|   IBIS model for TI xxx DSP
[IBIS Ver]   5.1
[Disclaimer]   Please be aware that in the absence of a written agreement
|   Texas Instruments(TI) assumes no liability for:
|   (1) The accuracy of the IBIS models provided to your company,
|   however, the IBIS model is compliant to industry standard
|   IQ Level 2a.  Refer to IBIS Quality Section below for
|   for full details.
|   (2) The proper functioning of these Models in your design
|   or for any resulting applications
|   (3) Infringement of patents, copyrights or intellectual
|   property rights resulting from your use of these
|   models.
|   TI provides IBIS Models as a service to our customers and
|   therefore reserves the right to limit distribution of the
|   Models.  The information is subject to change without notice.
[File Name]  j742s2.ibs
[File Rev]   0.1
|   -Initial version
[Date]   28 March 2024
[Source]   Texas Instruments Incorporated
[Copyright]   Property of Texas Instruments Incorporated.
|   Unauthorized reproduction and/or distribution is strictly.
|   prohibited.
|   This product is protected under copyright law and trade
|   secret law as an unpublished work.
|   Created 2012,(C) Copyright 1999-2012,
|   Texas Instruments Incorporated., All Rights Reserved.
|   These commodities are under the U.S. Government
|   distribution license control. As such,they are not to be
|   re-exported without the prior approval of the U.S.
|   Department of Commerce.
[Notes]
|   This file does not include AMI models for the following:
|   1. PCIe
|   2. CSI
|   3. Display Port
|   4. USB2
|   5. USB3
|   6. MPHY
|   For SerDes simulations use Texas Instruments IBIS AMI models
|   Some IV curves contain Non monotonic data points.
|   Revision History
|   GERNERAL COMMENT: All IBIS Quality Notes below reflect latest release
|   and version of IBIS File
|   File passes ibischk6 and ibischk7 with 0 errors and 91 warnings
|   v0.1: Initial version
|   Component j742s2
[Component] j742s2
[Manufacturer] Texas Instruments
[Package]
|   typ   min   max
R_pkg   0.61008   0.049437   1.2542
L_pkg   3.63e-9   6.144e-10   6.964e-9
C_pkg   1.799e-12   7.984e-13   3.865e-12
[Pin]	Signal_name	model_name
M30	ATEST0	NC
J29	ATEST1	NC
T27	CAP_VDDS0	POWER
J25	CAP_VDDS0_MCU	POWER
J23	CAP_VDDS1_MCU	POWER
P27	CAP_VDDS2	POWER
J24	CAP_VDDS2_MCU	POWER
M27	CAP_VDDS5	POWER
AH33	CSI0_RXCLKN	NC
AH32	CSI0_RXCLKP	NC
AL32	CSI0_RXN0	NC
AM31	CSI0_RXN1	NC
AN30	CSI0_RXN2	NC
AK33	CSI0_RXN3	NC
AL31	CSI0_RXP0	NC
AM30	CSI0_RXP1	NC
AN29	CSI0_RXP2	NC
AK32	CSI0_RXP3	NC
AH31	CSI0_RXRCALIB	NC
AE29	CSI1_RXCLKN	NC
AF29	CSI1_RXCLKP	NC
AF30	CSI1_RXN0	NC
AE33	CSI1_RXN1	NC
AE31	CSI1_RXN2	NC
AF32	CSI1_RXN3	NC
AG30	CSI1_RXP0	NC
AF33	CSI1_RXP1	NC
AF31	CSI1_RXP2	NC
AG32	CSI1_RXP3	NC
AJ33	CSI1_RXRCALIB	NC
AC29	CSI2_RXCLKN	NC
AB29	CSI2_RXCLKP	NC
AC30	CSI2_RXN0	NC
AB31	CSI2_RXN1	NC
AC32	CSI2_RXN2	NC
AB33	CSI2_RXN3	NC
AD30	CSI2_RXP0	NC
AC31	CSI2_RXP1	NC
AD32	CSI2_RXP2	NC
AC33	CSI2_RXP3	NC
AH29	CSI2_RXRCALIB	NC
AA3	DDR0_CA0	DDR_SE
Y4	DDR0_CA1	DDR_SE
AA4	DDR0_CA2	DDR_SE
AB3	DDR0_CA3	DDR_SE
Y3	DDR0_CA4	DDR_SE
AB5	DDR0_CA5	DDR_SE
R7	DDR0_CAL0	DDR_SE
AB6	DDR0_CKE0	DDR_SE
AB7	DDR0_CKE1	DDR_SE
Y2	DDR0_CKN	DDR_DIFF
AA1	DDR0_CKP	DDR_DIFF
AA6	DDR0_CSN0_0	DDR_SE
Y5	DDR0_CSN0_1	DDR_SE
Y7	DDR0_CSN1_0	DDR_SE
AA7	DDR0_CSN1_1	DDR_SE
U6	DDR0_DM0	DDR_SE
V2	DDR0_DM1	DDR_SE
AE2	DDR0_DM2	DDR_SE
AF6	DDR0_DM3	DDR_SE
R5	DDR0_DQ0	DDR_SE
R4	DDR0_DQ1	DDR_SE
W3	DDR0_DQ10	DDR_SE
V5	DDR0_DQ11	DDR_SE
W6	DDR0_DQ12	DDR_SE
U2	DDR0_DQ13	DDR_SE
W4	DDR0_DQ14	DDR_SE
U3	DDR0_DQ15	DDR_SE
AD5	DDR0_DQ16	DDR_SE
AC3	DDR0_DQ17	DDR_SE
AE3	DDR0_DQ18	DDR_SE
AB2	DDR0_DQ19	DDR_SE
R2	DDR0_DQ2	DDR_SE
AC4	DDR0_DQ20	DDR_SE
AD2	DDR0_DQ21	DDR_SE
AC6	DDR0_DQ22	DDR_SE
AD4	DDR0_DQ23	DDR_SE
AG4	DDR0_DQ24	DDR_SE
AG2	DDR0_DQ25	DDR_SE
AF3	DDR0_DQ26	DDR_SE
AE5	DDR0_DQ27	DDR_SE
AE6	DDR0_DQ28	DDR_SE
AG5	DDR0_DQ29	DDR_SE
T4	DDR0_DQ3	DDR_SE
AF4	DDR0_DQ30	DDR_SE
AH6	DDR0_DQ31	DDR_SE
U5	DDR0_DQ4	DDR_SE
T3	DDR0_DQ5	DDR_SE
T6	DDR0_DQ6	DDR_SE
T7	DDR0_DQ7	DDR_SE
V4	DDR0_DQ8	DDR_SE
V7	DDR0_DQ9	DDR_SE
T1	DDR0_DQS0N	DDR_DIFF
R1	DDR0_DQS0P	DDR_DIFF
W1	DDR0_DQS1N	DDR_DIFF
V1	DDR0_DQS1P	DDR_DIFF
AC1	DDR0_DQS2N	DDR_DIFF
AD1	DDR0_DQS2P	DDR_DIFF
AF1	DDR0_DQS3N	DDR_DIFF
AG1	DDR0_DQS3P	DDR_DIFF
W7	DDR0_RESETN	DDR_SE
AC7	DDR0_RET	DDR_SE
J4	DDR1_CA0	DDR_SE
H3	DDR1_CA1	DDR_SE
G2	DDR1_CA2	DDR_SE
J3	DDR1_CA3	DDR_SE
G3	DDR1_CA4	DDR_SE
H4	DDR1_CA5	DDR_SE
F8	DDR1_CAL0	DDR_SE
E7	DDR1_CKE0	DDR_SE
H6	DDR1_CKE1	DDR_SE
H1	DDR1_CKN	DDR_DIFF
J2	DDR1_CKP	DDR_DIFF
G6	DDR1_CSN0_0	DDR_SE
G7	DDR1_CSN0_1	DDR_SE
H7	DDR1_CSN1_0	DDR_SE
F6	DDR1_CSN1_1	DDR_SE
A3	DDR1_DM0	DDR_SE
F3	DDR1_DM1	DDR_SE
L2	DDR1_DM2	DDR_SE
P2	DDR1_DM3	DDR_SE
A6	DDR1_DQ0	DDR_SE
C6	DDR1_DQ1	DDR_SE
E2	DDR1_DQ10	DDR_SE
F4	DDR1_DQ11	DDR_SE
D6	DDR1_DQ12	DDR_SE
E4	DDR1_DQ13	DDR_SE
D3	DDR1_DQ14	DDR_SE
D5	DDR1_DQ15	DDR_SE
M3	DDR1_DQ16	DDR_SE
K4	DDR1_DQ17	DDR_SE
M2	DDR1_DQ18	DDR_SE
L5	DDR1_DQ19	DDR_SE
A5	DDR1_DQ2	DDR_SE
J5	DDR1_DQ20	DDR_SE
K3	DDR1_DQ21	DDR_SE
L4	DDR1_DQ22	DDR_SE
K6	DDR1_DQ23	DDR_SE
N6	DDR1_DQ24	DDR_SE
P4	DDR1_DQ25	DDR_SE
N3	DDR1_DQ26	DDR_SE
M5	DDR1_DQ27	DDR_SE
M6	DDR1_DQ28	DDR_SE
P5	DDR1_DQ29	DDR_SE
C4	DDR1_DQ3	DDR_SE
N4	DDR1_DQ30	DDR_SE
P6	DDR1_DQ31	DDR_SE
B4	DDR1_DQ4	DDR_SE
B2	DDR1_DQ5	DDR_SE
C3	DDR1_DQ6	DDR_SE
B5	DDR1_DQ7	DDR_SE
E5	DDR1_DQ8	DDR_SE
D2	DDR1_DQ9	DDR_SE
C1	DDR1_DQS0N	DDR_DIFF
B1	DDR1_DQS0P	DDR_DIFF
F1	DDR1_DQS1N	DDR_DIFF
E1	DDR1_DQS1P	DDR_DIFF
K1	DDR1_DQS2N	DDR_DIFF
L1	DDR1_DQS2P	DDR_DIFF
N1	DDR1_DQS3N	DDR_DIFF
P1	DDR1_DQS3P	DDR_DIFF
G5	DDR1_RESETN	DDR_SE
G8	DDR1_RET	DDR_SE
AJ25	DP0_AUXN	NC
AJ24	DP0_AUXP	NC
AJ28	DSI0_TXCLKN	NC
AJ27	DSI0_TXCLKP	NC
AL26	DSI0_TXN0	NC
AK27	DSI0_TXN1	NC
AM25	DSI0_TXN2	NC
AN24	DSI0_TXN3	NC
AL25	DSI0_TXP0	NC
AK26	DSI0_TXP1	NC
AM24	DSI0_TXP2	NC
AN23	DSI0_TXP3	NC
AH25	DSI0_TXRCALIB	NC
AJ31	DSI1_TXCLKN	NC
AJ30	DSI1_TXCLKP	NC
AK30	DSI1_TXN0	NC
AL29	DSI1_TXN1	NC
AM28	DSI1_TXN2	NC
AN27	DSI1_TXN3	NC
AK29	DSI1_TXP0	NC
AL28	DSI1_TXP1	NC
AM27	DSI1_TXP2	NC
AN26	DSI1_TXP3	NC
AH27	DSI1_TXRCALIB	NC
L31	ECAP0_IN_APWM_OUT	LVCMOS_H
F19	EMU0	LVCMOS_V
E17	EMU1	LVCMOS_V
J33	EXT_REFCLK1	LVCMOS_H
Y29	EXTINTN	IIC_H
P32	GPIO0_11	LVCMOS_H
E33	GPIO0_12	LVCMOS_H
AA30	I2C0_SCL	IIC_H
Y30	I2C0_SDA	IIC_H
L30	IFORCE	NC
AH7	LJCB_DUAL_ATEST0	NC
AH8	LJCB_DUAL_ATEST1	NC
L28	MAIN_ATEST	NC
G29	MCAN0_RX	LVCMOS_H
N33	MCAN0_TX	LVCMOS_H
H31	MCAN1_RX	LVCMOS_H
G33	MCAN1_TX	LVCMOS_H
T29	MCAN12_RX	LVCMOS_H
P29	MCAN12_TX	LVCMOS_H
T32	MCAN13_RX	LVCMOS_H
T31	MCAN13_TX	LVCMOS_H
R30	MCAN14_RX	LVCMOS_H
R33	MCAN14_TX	LVCMOS_H
R31	MCAN15_RX	LVCMOS_H
R29	MCAN15_TX	LVCMOS_H
U30	MCAN16_RX	LVCMOS_H
G30	MCAN16_TX	LVCMOS_H
F33	MCAN2_RX	LVCMOS_H
G28	MCAN2_TX	LVCMOS_H
J30	MCASP0_ACLKX	LVCMOS_H
K31	MCASP0_AFSX	LVCMOS_H
F32	MCASP0_AXR0	LVCMOS_H
H32	MCASP0_AXR1	LVCMOS_H
L32	MCASP0_AXR10	LVCMOS_H
P30	MCASP0_AXR11	LVCMOS_H
M32	MCASP0_AXR12	LVCMOS_H
L33	MCASP0_AXR13	LVCMOS_H
U31	MCASP0_AXR14	LVCMOS_H
M33	MCASP0_AXR15	LVCMOS_H
H33	MCASP0_AXR2	LVCMOS_H
F31	MCASP0_AXR3	LVCMOS_H
J32	MCASP0_AXR4	LVCMOS_H
H30	MCASP0_AXR5	LVCMOS_H
K33	MCASP0_AXR6	LVCMOS_H
M31	MCASP0_AXR7	LVCMOS_H
N30	MCASP0_AXR8	LVCMOS_H
T33	MCASP0_AXR9	LVCMOS_H
U32	MCASP1_ACLKX	LVCMOS_H
N32	MCASP1_AFSX	LVCMOS_H
H29	MCASP1_AXR0	LVCMOS_H
G31	MCASP1_AXR1	LVCMOS_H
J31	MCASP1_AXR2	LVCMOS_H
P31	MCASP1_AXR3	LVCMOS_H
N31	MCASP1_AXR4	LVCMOS_H
P33	MCASP2_ACLKX	LVCMOS_H
G32	MCASP2_AFSX	LVCMOS_H
K32	MCASP2_AXR0	LVCMOS_H
R32	MCASP2_AXR1	LVCMOS_H
E26	MCU_ADC0_AIN0	NC
F25	MCU_ADC0_AIN1	NC
F23	MCU_ADC0_AIN2	NC
A28	MCU_ADC0_AIN3	NC
E24	MCU_ADC0_AIN4	NC
D27	MCU_ADC0_AIN5	NC
A26	MCU_ADC0_AIN6	NC
B27	MCU_ADC0_AIN7	NC
C26	MCU_ADC0_REFN	NC
D25	MCU_ADC0_REFP	NC
C32	MCU_ADC1_AIN0	NC
B33	MCU_ADC1_AIN1	NC
B31	MCU_ADC1_AIN2	NC
B29	MCU_ADC1_AIN3	NC
D31	MCU_ADC1_AIN4	NC
A32	MCU_ADC1_AIN5	NC
A30	MCU_ADC1_AIN6	NC
C28	MCU_ADC1_AIN7	NC
D29	MCU_ADC1_REFN	NC
C30	MCU_ADC1_REFP	NC
D22	MCU_I2C0_SCL	IIC_V
A21	MCU_I2C0_SDA	IIC_V
C18	MCU_MCAN0_RX	LVCMOS_V
E22	MCU_MCAN0_TX	LVCMOS_V
E12	MCU_MDIO0_MDC	LVCMOS_V
F13	MCU_MDIO0_MDIO	LVCMOS_V
D8	MCU_OSPI0_CLK	LVCMOS_V
F12	MCU_OSPI0_CSN0	LVCMOS_V
F11	MCU_OSPI0_CSN1	LVCMOS_V
F10	MCU_OSPI0_CSN2	LVCMOS_V
E11	MCU_OSPI0_CSN3	LVCMOS_V
E10	MCU_OSPI0_D0	LVCMOS_V
F9	MCU_OSPI0_D1	LVCMOS_V
E9	MCU_OSPI0_D2	LVCMOS_V
D11	MCU_OSPI0_D3	LVCMOS_V
D9	MCU_OSPI0_D4	LVCMOS_V
C9	MCU_OSPI0_D5	LVCMOS_V
C7	MCU_OSPI0_D6	LVCMOS_V
C8	MCU_OSPI0_D7	LVCMOS_V
C10	MCU_OSPI0_DQS	LVCMOS_V
D10	MCU_OSPI0_LBCLKO	LVCMOS_V
B7	MCU_OSPI1_CLK	LVCMOS_V
A8	MCU_OSPI1_CSN0	LVCMOS_V
A9	MCU_OSPI1_CSN1	LVCMOS_V
B8	MCU_OSPI1_D0	LVCMOS_V
B11	MCU_OSPI1_D1	LVCMOS_V
A11	MCU_OSPI1_D2	LVCMOS_V
A10	MCU_OSPI1_D3	LVCMOS_V
B9	MCU_OSPI1_DQS	LVCMOS_V
B10	MCU_OSPI1_LBCLKO	LVCMOS_V
C24	MCU_PORZ	RESET_H
E21	MCU_RESETSTATZ	LVCMOS_V
E20	MCU_RESETZ	LVCMOS_V
E13	MCU_RGMII1_RD0	LVCMOS_V
D14	MCU_RGMII1_RD1	LVCMOS_V
D12	MCU_RGMII1_RD2	LVCMOS_V
D13	MCU_RGMII1_RD3	LVCMOS_V
C12	MCU_RGMII1_RX_CTL	LVCMOS_V
C14	MCU_RGMII1_RXC	LVCMOS_V
B13	MCU_RGMII1_TD0	LVCMOS_V
A13	MCU_RGMII1_TD1	LVCMOS_V
B12	MCU_RGMII1_TD2	LVCMOS_V
A12	MCU_RGMII1_TD3	LVCMOS_V
B14	MCU_RGMII1_TX_CTL	LVCMOS_V
A14	MCU_RGMII1_TXC	LVCMOS_V
C22	MCU_SAFETY_ERRORN	LVCMOS_V
F15	MCU_SPI0_CLK	LVCMOS_V
E19	MCU_SPI0_CS0	LVCMOS_V
E18	MCU_SPI0_D0	LVCMOS_V
E14	MCU_SPI0_D1	LVCMOS_V
AH2	MMC0_CALPAD	EMMC
AJ2	MMC0_CLK	EMMC
AL2	MMC0_CMD	EMMC
AM1	MMC0_DAT0	EMMC
AK3	MMC0_DAT1	EMMC
AL1	MMC0_DAT2	EMMC
AK1	MMC0_DAT3	EMMC
AJ3	MMC0_DAT4	EMMC
AH3	MMC0_DAT5	EMMC
AJ4	MMC0_DAT6	EMMC
AK2	MMC0_DAT7	EMMC
AJ1	MMC0_DS	EMMC
AH4	MMC0_VCTRL_TP	EMMC
D33	MMC1_CLK	SDIO_H
E32	MMC1_CMD	SDIO_H
F28	MMC1_DAT0	SDIO_H
F29	MMC1_DAT1	SDIO_H
E30	MMC1_DAT2	SDIO_H
F30	MMC1_DAT3	SDIO_H
B23	OSC1_XI	NC
A22	OSC1_XO	NC
AJ13	PCIE_REFCLK0_N_OUT	NC
AJ12	PCIE_REFCLK0_P_OUT	NC
AH14	PCIE_REFCLK1_N_OUT	NC
AH13	PCIE_REFCLK1_P_OUT	NC
AH11	PCIE_REFCLK2_N_OUT	NC
AH10	PCIE_REFCLK2_P_OUT	NC
AJ16	PCIE_REFCLK3_N_OUT	NC
AJ15	PCIE_REFCLK3_P_OUT	NC
B16	PMIC_POWER_EN1	LVCMOS_V
T30	PMIC_WAKE0	LVCMOS_H
D24	PORZ	RESET_H
G20	RESET_REQZ	LVCMOS_V
W32	RESETSTATZ	LVCMOS_H
AK15	SERDES0_REFCLK_N	NC
AK14	SERDES0_REFCLK_P	NC
AG7	SERDES0_REXT	NC
AM12	SERDES0_RX0_N	NC
AM13	SERDES0_RX0_P	NC
AL13	SERDES0_RX1_N	NC
AL14	SERDES0_RX1_P	NC
AN15	SERDES0_RX2_N	NC
AN14	SERDES0_RX2_P	NC
AL17	SERDES0_RX3_N	NC
AL16	SERDES0_RX3_P	NC
AN11	SERDES0_TX0_N	NC
AN12	SERDES0_TX0_P	NC
AJ19	SERDES0_TX1_N	NC
AJ18	SERDES0_TX1_P	NC
AM16	SERDES0_TX2_N	NC
AM15	SERDES0_TX2_P	NC
AK18	SERDES0_TX3_N	NC
AK17	SERDES0_TX3_P	NC
AN5	SERDES1_REFCLK_N	NC
AN6	SERDES1_REFCLK_P	NC
AH9	SERDES1_REXT	NC
AL10	SERDES1_RX0_N	NC
AL11	SERDES1_RX0_P	NC
AN8	SERDES1_RX1_N	NC
AN9	SERDES1_RX1_P	NC
AM6	SERDES1_RX2_N	NC
AM7	SERDES1_RX2_P	NC
AL7	SERDES1_RX3_N	NC
AL8	SERDES1_RX3_P	NC
AK11	SERDES1_TX0_N	NC
AK12	SERDES1_TX0_P	NC
AM9	SERDES1_TX1_N	NC
AM10	SERDES1_TX1_P	NC
AK8	SERDES1_TX2_N	NC
AK9	SERDES1_TX2_P	NC
AJ9	SERDES1_TX3_N	NC
AJ10	SERDES1_TX3_P	NC
AK21	SERDES4_REFCLK_N	NC
AK20	SERDES4_REFCLK_P	NC
AH23	SERDES4_REXT	NC
AN17	SERDES4_RX0_N	NC
AN18	SERDES4_RX0_P	NC
AL19	SERDES4_RX1_N	NC
AL20	SERDES4_RX1_P	NC
AK23	SERDES4_RX2_N	NC
AK24	SERDES4_RX2_P	NC
AM21	SERDES4_RX3_N	NC
AM22	SERDES4_RX3_P	NC
AJ21	SERDES4_TX0_N	NC
AJ22	SERDES4_TX0_P	NC
AM18	SERDES4_TX1_N	NC
AM19	SERDES4_TX1_P	NC
AN20	SERDES4_TX2_N	NC
AN21	SERDES4_TX2_P	NC
AL22	SERDES4_TX3_N	NC
AL23	SERDES4_TX3_P	NC
Y31	SOC_SAFETY_ERRORN	LVCMOS_H
V31	SPI0_CLK	LVCMOS_H
Y33	SPI0_CS0	LVCMOS_H
Y32	SPI0_CS1	LVCMOS_H
V30	SPI0_D0	LVCMOS_H
W31	SPI0_D1	LVCMOS_H
F21	TCK	LVCMOS_V
V33	TDI	LVCMOS_H
W33	TDO	LVCMOS_H
E28	TEMP_DIODE_P	NC
F27	TEMP_DIODE_P	NC
AA32	TIMER_IO0	LVCMOS_H
W30	TIMER_IO1	LVCMOS_H
V32	TMS	LVCMOS_H
F17	TRSTN	LVCMOS_V
AJ5	UFS0_REF_CLK	NC
AJ7	UFS0_RSTN	NC
AK5	UFS0_RX_DN0	NC
AL4	UFS0_RX_DN1	NC
AK6	UFS0_RX_DP0	NC
AL5	UFS0_RX_DP1	NC
AN2	UFS0_TX_DN0	NC
AM3	UFS0_TX_DN1	NC
AN3	UFS0_TX_DP0	NC
AM4	UFS0_TX_DP1	NC
AH16	USB0_DM	NC
AH17	USB0_DP	NC
AH20	USB0_ID	NC
AH22	USB0_RCALIB	NC
AG19	USB0_VBUS	NC
K9	VDD_CORE	POWER
K11	VDD_CORE	POWER
K15	VDD_CORE	POWER
K17	VDD_CORE	POWER
L10	VDD_CORE	POWER
L12	VDD_CORE	POWER
L14	VDD_CORE	POWER
L16	VDD_CORE	POWER
M9	VDD_CORE	POWER
M11	VDD_CORE	POWER
M13	VDD_CORE	POWER
M15	VDD_CORE	POWER
M17	VDD_CORE	POWER
N10	VDD_CORE	POWER
N12	VDD_CORE	POWER
N14	VDD_CORE	POWER
N16	VDD_CORE	POWER
N22	VDD_CORE	POWER
N24	VDD_CORE	POWER
N26	VDD_CORE	POWER
P9	VDD_CORE	POWER
P11	VDD_CORE	POWER
P25	VDD_CORE	POWER
R10	VDD_CORE	POWER
R22	VDD_CORE	POWER
R24	VDD_CORE	POWER
R26	VDD_CORE	POWER
T23	VDD_CORE	POWER
T25	VDD_CORE	POWER
U22	VDD_CORE	POWER
U24	VDD_CORE	POWER
U26	VDD_CORE	POWER
U28	VDD_CORE	POWER
V23	VDD_CORE	POWER
V27	VDD_CORE	POWER
W22	VDD_CORE	POWER
W24	VDD_CORE	POWER
W26	VDD_CORE	POWER
W28	VDD_CORE	POWER
Y23	VDD_CORE	POWER
Y27	VDD_CORE	POWER
AA24	VDD_CORE	POWER
AA26	VDD_CORE	POWER
AA28	VDD_CORE	POWER
AB23	VDD_CORE	POWER
AB25	VDD_CORE	POWER
AB27	VDD_CORE	POWER
AC22	VDD_CORE	POWER
AC24	VDD_CORE	POWER
AC26	VDD_CORE	POWER
AC28	VDD_CORE	POWER
AD11	VDD_CORE	POWER
AD15	VDD_CORE	POWER
AD17	VDD_CORE	POWER
AD21	VDD_CORE	POWER
AD23	VDD_CORE	POWER
AD25	VDD_CORE	POWER
AD27	VDD_CORE	POWER
AE10	VDD_CORE	POWER
AE12	VDD_CORE	POWER
AE14	VDD_CORE	POWER
AE16	VDD_CORE	POWER
AE18	VDD_CORE	POWER
AE20	VDD_CORE	POWER
AE22	VDD_CORE	POWER
AE24	VDD_CORE	POWER
AE28	VDD_CORE	POWER
AF19	VDD_CORE	POWER
H19	VDD_CPU	POWER
H21	VDD_CPU	POWER
J18	VDD_CPU	POWER
J20	VDD_CPU	POWER
L18	VDD_CPU	POWER
L20	VDD_CPU	POWER
M19	VDD_CPU	POWER
N18	VDD_CPU	POWER
N20	VDD_CPU	POWER
P15	VDD_CPU	POWER
P17	VDD_CPU	POWER
P19	VDD_CPU	POWER
P21	VDD_CPU	POWER
R12	VDD_CPU	POWER
R20	VDD_CPU	POWER
T9	VDD_CPU	POWER
T11	VDD_CPU	POWER
T17	VDD_CPU	POWER
T19	VDD_CPU	POWER
T21	VDD_CPU	POWER
U8	VDD_CPU	POWER
U10	VDD_CPU	POWER
U18	VDD_CPU	POWER
U20	VDD_CPU	POWER
V11	VDD_CPU	POWER
V19	VDD_CPU	POWER
V21	VDD_CPU	POWER
W8	VDD_CPU	POWER
W10	VDD_CPU	POWER
W12	VDD_CPU	POWER
W18	VDD_CPU	POWER
W20	VDD_CPU	POWER
Y9	VDD_CPU	POWER
Y17	VDD_CPU	POWER
Y19	VDD_CPU	POWER
Y21	VDD_CPU	POWER
AA8	VDD_CPU	POWER
AA10	VDD_CPU	POWER
AA12	VDD_CPU	POWER
AA20	VDD_CPU	POWER
AB9	VDD_CPU	POWER
AB11	VDD_CPU	POWER
AB13	VDD_CPU	POWER
AB15	VDD_CPU	POWER
AB17	VDD_CPU	POWER
AB19	VDD_CPU	POWER
AB21	VDD_CPU	POWER
AC8	VDD_CPU	POWER
AC12	VDD_CPU	POWER
AC14	VDD_CPU	POWER
AC16	VDD_CPU	POWER
AC18	VDD_CPU	POWER
AC20	VDD_CPU	POWER
AD9	VDD_CPU	POWER
J22	VDD_MCU	POWER
K21	VDD_MCU	POWER
K23	VDD_MCU	POWER
L24	VDD_MCU	POWER
M21	VDD_MCU	POWER
M23	VDD_MCU	POWER
M25	VDD_MCU	POWER
J26	VDD_MCU_WAKE1	POWER
R27	VDD_WAKE0	POWER
AG24	VDDA_0P8_CSIRX0_1	POWER
AG26	VDDA_0P8_CSIRX2	POWER
AD7	VDDA_0P8_DLL_MMC0	POWER
AG22	VDDA_0P8_DSITX	POWER
AG23	VDDA_0P8_DSITX_C	POWER
P8	VDDA_0P8_PLL_DDR0	POWER
J11	VDDA_0P8_PLL_DDR1	POWER
AF10	VDDA_0P8_SERDES_C0_1	POWER
AF13	VDDA_0P8_SERDES_C0_1	POWER
AE15	VDDA_0P8_SERDES_C4	POWER
AF16	VDDA_0P8_SERDES_C4	POWER
AF12	VDDA_0P8_SERDES0_1	POWER
AG10	VDDA_0P8_SERDES0_1	POWER
AG13	VDDA_0P8_SERDES0_1	POWER
AG15	VDDA_0P8_SERDES4	POWER
AG16	VDDA_0P8_SERDES4	POWER
AF9	VDDA_0P8_UFS	POWER
AG17	VDDA_0P8_USB	POWER
AF25	VDDA_1P8_CSIRX0_1	POWER
AF26	VDDA_1P8_CSIRX0_1	POWER
AF27	VDDA_1P8_CSIRX2	POWER
AG27	VDDA_1P8_CSIRX2	POWER
AF22	VDDA_1P8_DSITX	POWER
AF23	VDDA_1P8_DSITX	POWER
AG11	VDDA_1P8_SERDES0_1	POWER
AG12	VDDA_1P8_SERDES0_1	POWER
AG21	VDDA_1P8_SERDES2_4	POWER
AF15	VDDA_1P8_SERDES4	POWER
AG8	VDDA_1P8_UFS	POWER
AH19	VDDA_1P8_USB	POWER
AF17	VDDA_3P3_USB	POWER
J28	VDDA_ADC0	POWER
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[Diff_pin]	inv_pin	vdiff	tdelay_typ	tdelay_min	tdelay_max
AA1	Y2	NA	NA	NA	NA
R1	T1	NA	NA	NA	NA
V1	W1	NA	NA	NA	NA
AD1	AC1	NA	NA	NA	NA
AG1	AF1	NA	NA	NA	NA
J2	H1	NA	NA	NA	NA
B1	C1	NA	NA	NA	NA
E1	F1	NA	NA	NA	NA
L1	K1	NA	NA	NA	NA
P1	N1	NA	NA	NA	NA
|---------------- DDR -------------------
[Model Selector] DDR_SE
lpddr4_ocd_240p_240n  driver with 240 ohms pullup and 240 ohms pulldown strength
lpddr4_ocd_120p_120n  driver with 120 ohms pullup and 120 ohms pulldown strength
lpddr4_ocd_80p_80n  driver with 80 ohms pullup and 80 ohms pulldown strength
lpddr4_ocd_60p_60n  driver with 60 ohms pullup and 60 ohms pulldown strength
lpddr4_ocd_48p_48n  driver with 48 ohms pullup and 48 ohms pulldown strength
lpddr4_ocd_40p_40n  driver with 40 ohms pullup and 40 ohms pulldown strength
lpddr4_ocd_120pd_60p_40n  driver with 60/40 ohms pullup/pulldown 120 ohms aopd strength
lpddr4_ocd_120pd_48p_40n  driver with 48/40 ohms pullup/pulldown 120 ohms aopd strength
lpddr4_odt_240  240 ohm termination
lpddr4_odt_120  120 ohm termination
lpddr4_odt_80  80 ohm termination
lpddr4_odt_60  60 ohm termination
lpddr4_odt_48  48 ohm termination
lpddr4_odt_40  40 ohm termination
lpddr4_odt_off  open ohm termination
[Model Selector] DDR_DIFF
lpddr4_ocd_240p_240n_diff  driver with 240 ohms pullup and 240 ohms pulldown strength
lpddr4_ocd_120p_120n_diff  driver with 120 ohms pullup and 120 ohms pulldown strength
lpddr4_ocd_80p_80n_diff  driver with 80 ohms pullup and 80 ohms pulldown strength
lpddr4_ocd_60p_60n_diff  driver with 60 ohms pullup and 60 ohms pulldown strength
lpddr4_ocd_48p_48n_diff  driver with 48 ohms pullup and 48 ohms pulldown strength
lpddr4_ocd_40p_40n_diff  driver with 40 ohms pullup and 40 ohms pulldown strength
lpddr4_ocd_120pd_60p_40n_diff  driver with 60/40 ohms pullup/pulldown 120 ohms aopd strength
lpddr4_ocd_120pd_48p_40n_diff  driver with 48/40 ohms pullup/pulldown 120 ohms aopd strength
lpddr4_odt_240_diff  240 ohm termination
lpddr4_odt_120_diff  120 ohm termination
lpddr4_odt_80_diff  80 ohm termination
lpddr4_odt_60_diff  60 ohm termination
lpddr4_odt_48_diff  48 ohm termination
lpddr4_odt_40_diff  40 ohm termination
lpddr4_odt_off_diff  open ohm termination
|****************** SDIO
[Model Selector] SDIO_H
sdio1_r33_1p8_h PRWDWUWSWEWCDGSDIO_H@_R33_1p8_comment
sdio1_r33_3p3_h PRWDWUWSWEWCDGSDIO_H@_R33_3p3_comment
sdio1_r40_1p8_h PRWDWUWSWEWCDGSDIO_H@_R40_1p8_comment
sdio1_r40_3p3_h PRWDWUWSWEWCDGSDIO_H@_R40_3p3_comment
sdio1_r50_1p8_h PRWDWUWSWEWCDGSDIO_H@_R50_1p8_comment
sdio1_r50_3p3_h PRWDWUWSWEWCDGSDIO_H@_R50_3p3_comment
sdio1_r66_1p8_h PRWDWUWSWEWCDGSDIO_H@_R66_1p8_comment
sdio1_r66_3p3_h PRWDWUWSWEWCDGSDIO_H@_R66_3p3_comment
sdio1_utr33_1p8_h PRWDWUWSWEWCDGSDIO_H@_UT_R33_1p8_comment
sdio1_utr33_3p3_h PRWDWUWSWEWCDGSDIO_H@_UT_R33_3p3_comment
sdio1_utr40_1p8_h PRWDWUWSWEWCDGSDIO_H@_UT_R40_1p8_comment
sdio1_utr40_3p3_h PRWDWUWSWEWCDGSDIO_H@_UT_R40_3p3_comment
sdio1_utr50_1p8_h PRWDWUWSWEWCDGSDIO_H@_UT_R50_1p8_comment
sdio1_utr50_3p3_h PRWDWUWSWEWCDGSDIO_H@_UT_R50_3p3_comment
sdio1_utr66_1p8_h PRWDWUWSWEWCDGSDIO_H@_UT_R66_1p8_comment
sdio1_utr66_3p3_h PRWDWUWSWEWCDGSDIO_H@_UT_R66_3p3_comment
|********** LVCMOS
[Model Selector] LVCMOS_H
lvcmos1_nom_1p8_h PRWDWUWSWEWCDGLVCMOS_H@_Nom_1p8_comment
lvcmos1_nom_3p3_h PRWDWUWSWEWCDGLVCMOS_H@_Nom_3p3_comment
lvcmos1_slow_1p8_h PRWDWUWSWEWCDGLVCMOS_H@_Slow_1p8_comment
lvcmos1_slow_3p3_h PRWDWUWSWEWCDGLVCMOS_H@_Slow_3p3_comment
lvcmos1_fast_1p8_h PRWDWUWSWEWCDGLVCMOS_H@_Fast_1p8_comment
lvcmos1_fast_3p3_h PRWDWUWSWEWCDGLVCMOS_H@_Fast_3p3_comment
lvcmos1_utnom_1p8_h PRWDWUWSWEWCDGLVCMOS_H@_UT_Nom_1p8_comment
lvcmos1_utnom_3p3_h PRWDWUWSWEWCDGLVCMOS_H@_UT_Nom_3p3_comment
lvcmos1_utslow_1p8_h PRWDWUWSWEWCDGLVCMOS_H@_UT_Slow_1p8_comment
lvcmos1_utslow_3p3_h PRWDWUWSWEWCDGLVCMOS_H@_UT_Slow_3p3_comment
lvcmos1_utfast_1p8_h PRWDWUWSWEWCDGLVCMOS_H@_UT_Fast_1p8_comment
lvcmos1_utfast_3p3_h PRWDWUWSWEWCDGLVCMOS_H@_UT_Fast_3p3_comment
[Model Selector] LVCMOS_V
lvcmos0_nom_1p8_v PRWDWUWSWEWCDGLVCMOS_V@_Nom_1p8_comment
lvcmos0_nom_3p3_v PRWDWUWSWEWCDGLVCMOS_V@_Nom_3p3_comment
lvcmos0_slow_1p8_v PRWDWUWSWEWCDGLVCMOS_V@_Slow_1p8_comment
lvcmos0_slow_3p3_v PRWDWUWSWEWCDGLVCMOS_V@_Slow_3p3_comment
lvcmos0_fast_1p8_v PRWDWUWSWEWCDGLVCMOS_V@_Fast_1p8_comment
lvcmos0_fast_3p3_v PRWDWUWSWEWCDGLVCMOS_V@_Fast_3p3_comment
lvcmos0_utnom_1p8_v PRWDWUWSWEWCDGLVCMOS_V@_UT_Nom_1p8_comment
lvcmos0_utnom_3p3_v PRWDWUWSWEWCDGLVCMOS_V@_UT_Nom_3p3_comment
lvcmos0_utslow_1p8_v PRWDWUWSWEWCDGLVCMOS_V@_UT_Slow_1p8_comment
lvcmos0_utslow_3p3_v PRWDWUWSWEWCDGLVCMOS_V@_UT_Slow_3p3_comment
lvcmos0_utfast_1p8_v PRWDWUWSWEWCDGLVCMOS_V@_UT_Fast_1p8_comment
lvcmos0_utfast_3p3_v PRWDWUWSWEWCDGLVCMOS_V@_UT_Fast_3p3_comment
[Model Selector] IIC_H
Cell18_0_0_H PRBOPDDGZIIC_H@HSMODE_HSMCSE=0_0_comment 1.8V
Cell18_0_1_H PRBOPDDGZIIC_H@HSMODE_HSMCSE=0_1_comment 1.8V
Cell18_0_2_H PRBOPDDGZIIC_H@HSMODE_HSMCSE=1_0_comment 1.8V
Cell18_0_3_H PRBOPDDGZIIC_H@HSMODE_HSMCSE=1_1_comment 1.8V
Cell33_0_0_H PRBOPDDGZIIC_H@HSMODE_HSMCSE=0_0_comment
Cell33_0_1_H PRBOPDDGZIIC_H@HSMODE_HSMCSE=0_1_comment
Cell33_0_2_H PRBOPDDGZIIC_H@HSMODE_HSMCSE=1_0_comment
Cell33_0_3_H PRBOPDDGZIIC_H@HSMODE_HSMCSE=1_1_comment
[Model Selector] IIC_V
Cell18_1_0 PRBOPDDGZIIC_V@HSMODE_HSMCSE=0_0_comment  1.8V
Cell18_1_1 PRBOPDDGZIIC_V@HSMODE_HSMCSE=0_1_comment  1.8V
Cell18_1_2 PRBOPDDGZIIC_V@HSMODE_HSMCSE=1_0_comment  1.8V
Cell18_1_3 PRBOPDDGZIIC_V@HSMODE_HSMCSE=1_1_comment  1.8V
Cell33_1_0 PRBOPDDGZIIC_V@HSMODE_HSMCSE=0_0_comment
Cell33_1_1 PRBOPDDGZIIC_V@HSMODE_HSMCSE=0_1_comment
Cell33_1_2 PRBOPDDGZIIC_V@HSMODE_HSMCSE=1_0_comment
Cell33_1_3 PRBOPDDGZIIC_V@HSMODE_HSMCSE=1_1_comment
|***************** RESET ************************************************
[Model Selector] RESET_H
reset18_0_0 PDIDGZRESET_H
|   EMMC
[MODEL SELECTOR] EMMC
emmc51_io_tx33ohm   33ohm DRIVER
emmc51_io_tx40ohm   40ohm DRIVER
emmc51_io_tx50ohm   50ohm DRIVER
emmc51_io_tx66ohm   66ohm DRIVER
emmc51_io_tx100ohm  100ohm DRIVER
emmc51_io_txod   Open drain DRIVER
|******************** Package Model *************************************
[Define Package Model]   j742s2_pkg
[Manufacturer]   Texas Instruments
[OEM]   name 2
[Description]   533-pin Package
|[Number of Sections]   1
[Number of Pins]   533
[Pin Numbers]
|[Pin Name]  Net Number   Net Name   Net's All Pins
T27   | 1   CAP_VDDS0   T27
J25   | 2   CAP_VDDS0_MCU   J25
J23   | 3   CAP_VDDS1_MCU   J23
P27   | 4   CAP_VDDS2   P27
J24   | 5   CAP_VDDS2_MCU   J24
M27   | 6   CAP_VDDS5   M27
AA22   | 7   VDDAR_CORE   AA22
   |AD13
   |AD16
   |AD19
   |AE9
   |AE26
   |P23
   |Y25
AA14   | 8   VDDAR_CPU   AA14
   |AA16
   |AA18
   |AC10
   |K19
   |L21
   |P13
   |R18
   |U12
   |U19
   |V9
   |V17
   |Y11
K25   | 9   VDDAR_MCU   K25
   |L22
AG24   | 10   VDDA_0P8_CSIRX0_1   AG24
AG26   | 11   VDDA_0P8_CSIRX2   AG26
AD7   | 12   VDDA_0P8_DLL_MMC0   AD7
AG22   | 13   VDDA_0P8_DSITX   AG22
AG23   | 14   VDDA_0P8_DSITX_C   AG23
P8   | 15   VDDA_0P8_PLL_DDR0   P8
J11   | 16   VDDA_0P8_PLL_DDR1   J11
AF12   | 17   VDDA_0P8_SERDES0_1   AF12
   |AG10
   |AG13
AG15   | 18   VDDA_0P8_SERDES4   AG15
   |AG16
AF10   | 19   VDDA_0P8_SERDES_C0_1   AF10
   |AF13
AE15   | 20   VDDA_0P8_SERDES_C4   AE15
   |AF16
AF9   | 21   VDDA_0P8_UFS   AF9
AG17   | 22   VDDA_0P8_USB   AG17
AF25   | 23   VDDA_1P8_CSIRX0_1   AF25
   |AF26
AF27   | 24   VDDA_1P8_CSIRX2   AF27
   |AG27
AF22   | 25   VDDA_1P8_DSITX   AF22
   |AF23
AG11   | 26   VDDA_1P8_SERDES0_1   AG11
   |AG12
AG21   | 27   VDDA_1P8_SERDES2_4   AG21
AF15   | 28   VDDA_1P8_SERDES4   AF15
AG8   | 29   VDDA_1P8_UFS   AG8
AH19   | 30   VDDA_1P8_USB   AH19
AF17   | 31   VDDA_3P3_USB   AF17
J28   | 32   VDDA_ADC0   J28
K28   | 33   VDDA_ADC1   K28
K26   | 34   VDDA_MCU_PLLGRP0   K26
K24   | 35   VDDA_MCU_TEMP   K24
L27   | 36   VDDA_OSC1   L27
W25   | 37   VDDA_PLLGRP0   W25
V25   | 38   VDDA_PLLGRP1   V25
AE11   | 39   VDDA_PLLGRP2   AE11
T12   | 40   VDDA_PLLGRP5   T12
N19   | 41   VDDA_PLLGRP6   N19
M10   | 42   VDDA_PLLGRP7   M10
K13   | 43   VDDA_PLLGRP8   K13
V24   | 44   VDDA_PLLGRP9   V24
AD20   | 45   VDDA_PLLGRP10   AD20
W21   | 46   VDDA_PLLGRP12   W21
Y24   | 47   VDDA_PLLGRP13   Y24
L26   | 48   VDDA_POR_WKUP   L26
V26   | 49   VDDA_TEMP0   V26
K10   | 50   VDDA_TEMP1   K10
U21   | 51   VDDA_TEMP2   U21
AC11   | 52   VDDA_TEMP3   AC11
AB16   | 53   VDDA_TEMP4   AB16
J27   | 54   VDDA_WKUP   J27
T28   | 55   VDDSHV0   T28
H27   | 56   VDDSHV0_MCU   H27
G22   | 57   VDDSHV1_MCU   G22
   |H23
N28   | 58   VDDSHV2   N28
   |P28
G24   | 59   VDDSHV2_MCU   G24
   |H25
N27   | 60   VDDSHV5   N27
A2   | 61   VDDS_DDR   A2
   |AH1
   |G10
   |G12
   |G14
   |G16
   |G18
   |H9
   |H11
   |H13
   |H15
   |H17
   |J8
   |J10
   |J14
   |J16
   |K7
   |L8
   |M7
   |P7
   |R8
N8   | 62   VDDS_DDR_C0   N8
J12   | 63   VDDS_DDR_C1   J12
AE8   | 64   VDDS_MMC0   AE8
   |AF7
AA24   | 65   VDD_CORE   AA24
   |AA26
   |AA28
   |AB23
   |AB25
   |AB27
   |AC22
   |AC24
   |AC26
   |AC28
   |AD11
   |AD15
   |AD17
   |AD21
   |AD23
   |AD25
   |AD27
   |AE10
   |AE12
   |AE14
   |AE16
   |AE18
   |AE20
   |AE22
   |AE24
   |AE28
   |AF19
   |K9
   |K11
   |K15
   |K17
   |L10
   |L12
   |L14
   |L16
   |M9
   |M11
   |M13
   |M15
   |M17
   |N10
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AA8   | 66   VDD_CPU   AA8
   |AA10
   |AA12
   |AA20
   |AB9
   |AB11
   |AB13
   |AB15
   |AB17
   |AB19
   |AB21
   |AC8
   |AC12
   |AC14
   |AC16
   |AC18
   |AC20
   |AD9
   |H19
   |H21
   |J18
   |J20
   |L18
   |L20
   |M19
   |N18
   |N20
   |P15
   |P17
   |P19
   |P21
   |R12
   |R20
   |T9
   |T11
   |T17
   |T19
   |T21
   |U8
   |U10
   |U18
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J22   | 67   VDD_MCU   J22
   |K21
   |K23
   |L24
   |M21
   |M23
   |M25
J26   | 68   VDD_MCU_WAKE1   J26
R27   | 69   VDD_WAKE0   R27
V29   | 70   VPP_CORE   V29
F26   | 71   VPP_MCU   F26
M30   | 72   ATEST0   M30
J29   | 73   ATEST1   J29
AH33   | 74   CSI0_RXCLKN   AH33
AH32   | 75   CSI0_RXCLKP   AH32
AL32   | 76   CSI0_RXN0   AL32
AM31   | 77   CSI0_RXN1   AM31
AN30   | 78   CSI0_RXN2   AN30
AK33   | 79   CSI0_RXN3   AK33
AL31   | 80   CSI0_RXP0   AL31
AM30   | 81   CSI0_RXP1   AM30
AN29   | 82   CSI0_RXP2   AN29
AK32   | 83   CSI0_RXP3   AK32
AH31   | 84   CSI0_RXRCALIB   AH31
AE29   | 85   CSI1_RXCLKN   AE29
AF29   | 86   CSI1_RXCLKP   AF29
AF30   | 87   CSI1_RXN0   AF30
AE33   | 88   CSI1_RXN1   AE33
AE31   | 89   CSI1_RXN2   AE31
AF32   | 90   CSI1_RXN3   AF32
AG30   | 91   CSI1_RXP0   AG30
AF33   | 92   CSI1_RXP1   AF33
AF31   | 93   CSI1_RXP2   AF31
AG32   | 94   CSI1_RXP3   AG32
AJ33   | 95   CSI1_RXRCALIB   AJ33
AC29   | 96   CSI2_RXCLKN   AC29
AB29   | 97   CSI2_RXCLKP   AB29
AC30   | 98   CSI2_RXN0   AC30
AB31   | 99   CSI2_RXN1   AB31
AC32   | 100   CSI2_RXN2   AC32
AB33   | 101   CSI2_RXN3   AB33
AD30   | 102   CSI2_RXP0   AD30
AC31   | 103   CSI2_RXP1   AC31
AD32   | 104   CSI2_RXP2   AD32
AC33   | 105   CSI2_RXP3   AC33
AH29   | 106   CSI2_RXRCALIB   AH29
AA3   | 107   DDR0_CA0   AA3
Y4   | 108   DDR0_CA1   Y4
AA4   | 109   DDR0_CA2   AA4
AB3   | 110   DDR0_CA3   AB3
Y3   | 111   DDR0_CA4   Y3
AB5   | 112   DDR0_CA5   AB5
R7   | 113   DDR0_CAL0   R7
AB6   | 114   DDR0_CKE0   AB6
AB7   | 115   DDR0_CKE1   AB7
Y2   | 116   DDR0_CKN   Y2
AA1   | 117   DDR0_CKP   AA1
AA6   | 118   DDR0_CSN0_0   AA6
Y5   | 119   DDR0_CSN0_1   Y5
Y7   | 120   DDR0_CSN1_0   Y7
AA7   | 121   DDR0_CSN1_1   AA7
U6   | 122   DDR0_DM0   U6
V2   | 123   DDR0_DM1   V2
AE2   | 124   DDR0_DM2   AE2
AF6   | 125   DDR0_DM3   AF6
R5   | 126   DDR0_DQ0   R5
R4   | 127   DDR0_DQ1   R4
R2   | 128   DDR0_DQ2   R2
T4   | 129   DDR0_DQ3   T4
U5   | 130   DDR0_DQ4   U5
T3   | 131   DDR0_DQ5   T3
T6   | 132   DDR0_DQ6   T6
T7   | 133   DDR0_DQ7   T7
V4   | 134   DDR0_DQ8   V4
V7   | 135   DDR0_DQ9   V7
W3   | 136   DDR0_DQ10   W3
V5   | 137   DDR0_DQ11   V5
W6   | 138   DDR0_DQ12   W6
U2   | 139   DDR0_DQ13   U2
W4   | 140   DDR0_DQ14   W4
U3   | 141   DDR0_DQ15   U3
AD5   | 142   DDR0_DQ16   AD5
AC3   | 143   DDR0_DQ17   AC3
AE3   | 144   DDR0_DQ18   AE3
AB2   | 145   DDR0_DQ19   AB2
AC4   | 146   DDR0_DQ20   AC4
AD2   | 147   DDR0_DQ21   AD2
AC6   | 148   DDR0_DQ22   AC6
AD4   | 149   DDR0_DQ23   AD4
AG4   | 150   DDR0_DQ24   AG4
AG2   | 151   DDR0_DQ25   AG2
AF3   | 152   DDR0_DQ26   AF3
AE5   | 153   DDR0_DQ27   AE5
AE6   | 154   DDR0_DQ28   AE6
AG5   | 155   DDR0_DQ29   AG5
AF4   | 156   DDR0_DQ30   AF4
AH6   | 157   DDR0_DQ31   AH6
T1   | 158   DDR0_DQS0N   T1
R1   | 159   DDR0_DQS0P   R1
W1   | 160   DDR0_DQS1N   W1
V1   | 161   DDR0_DQS1P   V1
AC1   | 162   DDR0_DQS2N   AC1
AD1   | 163   DDR0_DQS2P   AD1
AF1   | 164   DDR0_DQS3N   AF1
AG1   | 165   DDR0_DQS3P   AG1
W7   | 166   DDR0_RESETN   W7
AC7   | 167   DDR0_RET   AC7
J4   | 168   DDR1_CA0   J4
H3   | 169   DDR1_CA1   H3
G2   | 170   DDR1_CA2   G2
J3   | 171   DDR1_CA3   J3
G3   | 172   DDR1_CA4   G3
H4   | 173   DDR1_CA5   H4
F8   | 174   DDR1_CAL0   F8
E7   | 175   DDR1_CKE0   E7
H6   | 176   DDR1_CKE1   H6
H1   | 177   DDR1_CKN   H1
J2   | 178   DDR1_CKP   J2
G6   | 179   DDR1_CSN0_0   G6
G7   | 180   DDR1_CSN0_1   G7
H7   | 181   DDR1_CSN1_0   H7
F6   | 182   DDR1_CSN1_1   F6
A3   | 183   DDR1_DM0   A3
F3   | 184   DDR1_DM1   F3
L2   | 185   DDR1_DM2   L2
P2   | 186   DDR1_DM3   P2
A6   | 187   DDR1_DQ0   A6
C6   | 188   DDR1_DQ1   C6
A5   | 189   DDR1_DQ2   A5
C4   | 190   DDR1_DQ3   C4
B4   | 191   DDR1_DQ4   B4
B2   | 192   DDR1_DQ5   B2
C3   | 193   DDR1_DQ6   C3
B5   | 194   DDR1_DQ7   B5
E5   | 195   DDR1_DQ8   E5
D2   | 196   DDR1_DQ9   D2
E2   | 197   DDR1_DQ10   E2
F4   | 198   DDR1_DQ11   F4
D6   | 199   DDR1_DQ12   D6
E4   | 200   DDR1_DQ13   E4
D3   | 201   DDR1_DQ14   D3
D5   | 202   DDR1_DQ15   D5
M3   | 203   DDR1_DQ16   M3
K4   | 204   DDR1_DQ17   K4
M2   | 205   DDR1_DQ18   M2
L5   | 206   DDR1_DQ19   L5
J5   | 207   DDR1_DQ20   J5
K3   | 208   DDR1_DQ21   K3
L4   | 209   DDR1_DQ22   L4
K6   | 210   DDR1_DQ23   K6
N6   | 211   DDR1_DQ24   N6
P4   | 212   DDR1_DQ25   P4
N3   | 213   DDR1_DQ26   N3
M5   | 214   DDR1_DQ27   M5
M6   | 215   DDR1_DQ28   M6
P5   | 216   DDR1_DQ29   P5
N4   | 217   DDR1_DQ30   N4
P6   | 218   DDR1_DQ31   P6
C1   | 219   DDR1_DQS0N   C1
B1   | 220   DDR1_DQS0P   B1
F1   | 221   DDR1_DQS1N   F1
E1   | 222   DDR1_DQS1P   E1
K1   | 223   DDR1_DQS2N   K1
L1   | 224   DDR1_DQS2P   L1
N1   | 225   DDR1_DQS3N   N1
P1   | 226   DDR1_DQS3P   P1
G5   | 227   DDR1_RESETN   G5
G8   | 228   DDR1_RET   G8
AJ25   | 229   DP0_AUXN   AJ25
AJ24   | 230   DP0_AUXP   AJ24
AJ28   | 231   DSI0_TXCLKN   AJ28
AJ27   | 232   DSI0_TXCLKP   AJ27
AL26   | 233   DSI0_TXN0   AL26
AK27   | 234   DSI0_TXN1   AK27
AM25   | 235   DSI0_TXN2   AM25
AN24   | 236   DSI0_TXN3   AN24
AL25   | 237   DSI0_TXP0   AL25
AK26   | 238   DSI0_TXP1   AK26
AM24   | 239   DSI0_TXP2   AM24
AN23   | 240   DSI0_TXP3   AN23
AH25   | 241   DSI0_TXRCALIB   AH25
AJ31   | 242   DSI1_TXCLKN   AJ31
AJ30   | 243   DSI1_TXCLKP   AJ30
AK30   | 244   DSI1_TXN0   AK30
AL29   | 245   DSI1_TXN1   AL29
AM28   | 246   DSI1_TXN2   AM28
AN27   | 247   DSI1_TXN3   AN27
AK29   | 248   DSI1_TXP0   AK29
AL28   | 249   DSI1_TXP1   AL28
AM27   | 250   DSI1_TXP2   AM27
AN26   | 251   DSI1_TXP3   AN26
AH27   | 252   DSI1_TXRCALIB   AH27
L31   | 253   ECAP0_IN_APWM_OUT   L31
F19   | 254   EMU0   F19
E17   | 255   EMU1   E17
Y29   | 256   EXTINTN   Y29
J33   | 257   EXT_REFCLK1   J33
P32   | 258   GPIO0_11   P32
E33   | 259   GPIO0_12   E33
AA30   | 260   I2C0_SCL   AA30
Y30   | 261   I2C0_SDA   Y30
L30   | 262   IFORCE   L30
AH7   | 263   LJCB_DUAL_ATEST0   AH7
AH8   | 264   LJCB_DUAL_ATEST1   AH8
L28   | 265   MAIN_ATEST   L28
G29   | 266   MCAN0_RX   G29
N33   | 267   MCAN0_TX   N33
H31   | 268   MCAN1_RX   H31
G33   | 269   MCAN1_TX   G33
F33   | 270   MCAN2_RX   F33
G28   | 271   MCAN2_TX   G28
T29   | 272   MCAN12_RX   T29
P29   | 273   MCAN12_TX   P29
T32   | 274   MCAN13_RX   T32
T31   | 275   MCAN13_TX   T31
R30   | 276   MCAN14_RX   R30
R33   | 277   MCAN14_TX   R33
R31   | 278   MCAN15_RX   R31
R29   | 279   MCAN15_TX   R29
U30   | 280   MCAN16_RX   U30
G30   | 281   MCAN16_TX   G30
J30   | 282   MCASP0_ACLKX   J30
K31   | 283   MCASP0_AFSX   K31
F32   | 284   MCASP0_AXR0   F32
H32   | 285   MCASP0_AXR1   H32
H33   | 286   MCASP0_AXR2   H33
F31   | 287   MCASP0_AXR3   F31
J32   | 288   MCASP0_AXR4   J32
H30   | 289   MCASP0_AXR5   H30
K33   | 290   MCASP0_AXR6   K33
M31   | 291   MCASP0_AXR7   M31
N30   | 292   MCASP0_AXR8   N30
T33   | 293   MCASP0_AXR9   T33
L32   | 294   MCASP0_AXR10   L32
P30   | 295   MCASP0_AXR11   P30
M32   | 296   MCASP0_AXR12   M32
L33   | 297   MCASP0_AXR13   L33
U31   | 298   MCASP0_AXR14   U31
M33   | 299   MCASP0_AXR15   M33
U32   | 300   MCASP1_ACLKX   U32
N32   | 301   MCASP1_AFSX   N32
H29   | 302   MCASP1_AXR0   H29
G31   | 303   MCASP1_AXR1   G31
J31   | 304   MCASP1_AXR2   J31
P31   | 305   MCASP1_AXR3   P31
N31   | 306   MCASP1_AXR4   N31
P33   | 307   MCASP2_ACLKX   P33
G32   | 308   MCASP2_AFSX   G32
K32   | 309   MCASP2_AXR0   K32
R32   | 310   MCASP2_AXR1   R32
E26   | 311   MCU_ADC0_AIN0   E26
F25   | 312   MCU_ADC0_AIN1   F25
F23   | 313   MCU_ADC0_AIN2   F23
A28   | 314   MCU_ADC0_AIN3   A28
E24   | 315   MCU_ADC0_AIN4   E24
D27   | 316   MCU_ADC0_AIN5   D27
A26   | 317   MCU_ADC0_AIN6   A26
B27   | 318   MCU_ADC0_AIN7   B27
C26   | 319   MCU_ADC0_REFN   C26
D25   | 320   MCU_ADC0_REFP   D25
C32   | 321   MCU_ADC1_AIN0   C32
B33   | 322   MCU_ADC1_AIN1   B33
B31   | 323   MCU_ADC1_AIN2   B31
B29   | 324   MCU_ADC1_AIN3   B29
D31   | 325   MCU_ADC1_AIN4   D31
A32   | 326   MCU_ADC1_AIN5   A32
A30   | 327   MCU_ADC1_AIN6   A30
C28   | 328   MCU_ADC1_AIN7   C28
D29   | 329   MCU_ADC1_REFN   D29
C30   | 330   MCU_ADC1_REFP   C30
D22   | 331   MCU_I2C0_SCL   D22
A21   | 332   MCU_I2C0_SDA   A21
C18   | 333   MCU_MCAN0_RX   C18
E22   | 334   MCU_MCAN0_TX   E22
E12   | 335   MCU_MDIO0_MDC   E12
F13   | 336   MCU_MDIO0_MDIO   F13
D8   | 337   MCU_OSPI0_CLK   D8
F12   | 338   MCU_OSPI0_CSN0   F12
F11   | 339   MCU_OSPI0_CSN1   F11
F10   | 340   MCU_OSPI0_CSN2   F10
E11   | 341   MCU_OSPI0_CSN3   E11
E10   | 342   MCU_OSPI0_D0   E10
F9   | 343   MCU_OSPI0_D1   F9
E9   | 344   MCU_OSPI0_D2   E9
D11   | 345   MCU_OSPI0_D3   D11
D9   | 346   MCU_OSPI0_D4   D9
C9   | 347   MCU_OSPI0_D5   C9
C7   | 348   MCU_OSPI0_D6   C7
C8   | 349   MCU_OSPI0_D7   C8
C10   | 350   MCU_OSPI0_DQS   C10
D10   | 351   MCU_OSPI0_LBCLKO   D10
B7   | 352   MCU_OSPI1_CLK   B7
A8   | 353   MCU_OSPI1_CSN0   A8
A9   | 354   MCU_OSPI1_CSN1   A9
B8   | 355   MCU_OSPI1_D0   B8
B11   | 356   MCU_OSPI1_D1   B11
A11   | 357   MCU_OSPI1_D2   A11
A10   | 358   MCU_OSPI1_D3   A10
B9   | 359   MCU_OSPI1_DQS   B9
B10   | 360   MCU_OSPI1_LBCLKO   B10
C24   | 361   MCU_PORZ   C24
E21   | 362   MCU_RESETSTATZ   E21
E20   | 363   MCU_RESETZ   E20
E13   | 364   MCU_RGMII1_RD0   E13
D14   | 365   MCU_RGMII1_RD1   D14
D12   | 366   MCU_RGMII1_RD2   D12
D13   | 367   MCU_RGMII1_RD3   D13
C14   | 368   MCU_RGMII1_RXC   C14
C12   | 369   MCU_RGMII1_RX_CTL   C12
B13   | 370   MCU_RGMII1_TD0   B13
A13   | 371   MCU_RGMII1_TD1   A13
B12   | 372   MCU_RGMII1_TD2   B12
A12   | 373   MCU_RGMII1_TD3   A12
A14   | 374   MCU_RGMII1_TXC   A14
B14   | 375   MCU_RGMII1_TX_CTL   B14
C22   | 376   MCU_SAFETY_ERRORN   C22
F15   | 377   MCU_SPI0_CLK   F15
E19   | 378   MCU_SPI0_CS0   E19
E18   | 379   MCU_SPI0_D0   E18
E14   | 380   MCU_SPI0_D1   E14
AH2   | 381   MMC0_CALPAD   AH2
AJ2   | 382   MMC0_CLK   AJ2
AL2   | 383   MMC0_CMD   AL2
AM1   | 384   MMC0_DAT0   AM1
AK3   | 385   MMC0_DAT1   AK3
AL1   | 386   MMC0_DAT2   AL1
AK1   | 387   MMC0_DAT3   AK1
AJ3   | 388   MMC0_DAT4   AJ3
AH3   | 389   MMC0_DAT5   AH3
AJ4   | 390   MMC0_DAT6   AJ4
AK2   | 391   MMC0_DAT7   AK2
AJ1   | 392   MMC0_DS   AJ1
AH4   | 393   MMC0_VCTRL_TP   AH4
D33   | 394   MMC1_CLK   D33
E32   | 395   MMC1_CMD   E32
F28   | 396   MMC1_DAT0   F28
F29   | 397   MMC1_DAT1   F29
E30   | 398   MMC1_DAT2   E30
F30   | 399   MMC1_DAT3   F30
B23   | 400   OSC1_XI   B23
A22   | 401   OSC1_XO   A22
AJ13   | 402   PCIE_REFCLK0_N_OUT   AJ13
AJ12   | 403   PCIE_REFCLK0_P_OUT   AJ12
AH14   | 404   PCIE_REFCLK1_N_OUT   AH14
AH13   | 405   PCIE_REFCLK1_P_OUT   AH13
AH11   | 406   PCIE_REFCLK2_N_OUT   AH11
AH10   | 407   PCIE_REFCLK2_P_OUT   AH10
AJ16   | 408   PCIE_REFCLK3_N_OUT   AJ16
AJ15   | 409   PCIE_REFCLK3_P_OUT   AJ15
B16   | 410   PMIC_POWER_EN1   B16
T30   | 411   PMIC_WAKE0   T30
D24   | 412   PORZ   D24
W32   | 413   RESETSTATZ   W32
G20   | 414   RESET_REQZ   G20
AK15   | 415   SERDES0_REFCLK_N   AK15
AK14   | 416   SERDES0_REFCLK_P   AK14
AG7   | 417   SERDES0_REXT   AG7
AM12   | 418   SERDES0_RX0_N   AM12
AM13   | 419   SERDES0_RX0_P   AM13
AL13   | 420   SERDES0_RX1_N   AL13
AL14   | 421   SERDES0_RX1_P   AL14
AN15   | 422   SERDES0_RX2_N   AN15
AN14   | 423   SERDES0_RX2_P   AN14
AL17   | 424   SERDES0_RX3_N   AL17
AL16   | 425   SERDES0_RX3_P   AL16
AN11   | 426   SERDES0_TX0_N   AN11
AN12   | 427   SERDES0_TX0_P   AN12
AJ19   | 428   SERDES0_TX1_N   AJ19
AJ18   | 429   SERDES0_TX1_P   AJ18
AM16   | 430   SERDES0_TX2_N   AM16
AM15   | 431   SERDES0_TX2_P   AM15
AK18   | 432   SERDES0_TX3_N   AK18
AK17   | 433   SERDES0_TX3_P   AK17
AN5   | 434   SERDES1_REFCLK_N   AN5
AN6   | 435   SERDES1_REFCLK_P   AN6
AH9   | 436   SERDES1_REXT   AH9
AL10   | 437   SERDES1_RX0_N   AL10
AL11   | 438   SERDES1_RX0_P   AL11
AN8   | 439   SERDES1_RX1_N   AN8
AN9   | 440   SERDES1_RX1_P   AN9
AM6   | 441   SERDES1_RX2_N   AM6
AM7   | 442   SERDES1_RX2_P   AM7
AL7   | 443   SERDES1_RX3_N   AL7
AL8   | 444   SERDES1_RX3_P   AL8
AK11   | 445   SERDES1_TX0_N   AK11
AK12   | 446   SERDES1_TX0_P   AK12
AM9   | 447   SERDES1_TX1_N   AM9
AM10   | 448   SERDES1_TX1_P   AM10
AK8   | 449   SERDES1_TX2_N   AK8
AK9   | 450   SERDES1_TX2_P   AK9
AJ9   | 451   SERDES1_TX3_N   AJ9
AJ10   | 452   SERDES1_TX3_P   AJ10
AK21   | 453   SERDES4_REFCLK_N   AK21
AK20   | 454   SERDES4_REFCLK_P   AK20
AH23   | 455   SERDES4_REXT   AH23
AN17   | 456   SERDES4_RX0_N   AN17
AN18   | 457   SERDES4_RX0_P   AN18
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[Model Data]
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[End Model Data]
[End Package Model]
| Models and submodels in the file (93): lvcmos1_nom_1p8_h (I/O), lvcmos0_nom_1p8_v (I/O), lvcmos1_nom_3p3_h (I/O), lvcmos0_nom_3p3_v (I/O), lvcmos1_slow_1p8_h (I/O), lvcmos0_slow_1p8_v (I/O), lvcmos1_slow_3p3_h (I/O), lvcmos0_slow_3p3_v (I/O), lvcmos1_fast_1p8_h (I/O), lvcmos0_fast_1p8_v (I/O), lvcmos1_fast_3p3_h (I/O), lvcmos0_fast_3p3_v (I/O), lvcmos1_utnom_1p8_h (I/O), lvcmos0_utnom_1p8_v (I/O), lvcmos1_utnom_3p3_h (I/O), lvcmos0_utnom_3p3_v (I/O), lvcmos1_utslow_1p8_h (I/O), lvcmos0_utslow_1p8_v (I/O), lvcmos1_utslow_3p3_h (I/O), lvcmos0_utslow_3p3_v (I/O), lvcmos1_utfast_1p8_h (I/O), lvcmos0_utfast_1p8_v (I/O), lvcmos1_utfast_3p3_h (I/O), lvcmos0_utfast_3p3_v (I/O), sdio1_r33_1p8_h (I/O), sdio1_r33_3p3_h (I/O), sdio1_r40_1p8_h (I/O), sdio1_r40_3p3_h (I/O), sdio1_r50_1p8_h (I/O), sdio1_r50_3p3_h (I/O), sdio1_r66_1p8_h (I/O), sdio1_r66_3p3_h (I/O), sdio1_utr33_1p8_h (I/O), sdio1_utr33_3p3_h (I/O), sdio1_utr40_1p8_h (I/O), sdio1_utr40_3p3_h (I/O), sdio1_utr50_1p8_h (I/O), sdio1_utr50_3p3_h (I/O), sdio1_utr66_1p8_h (I/O), sdio1_utr66_3p3_h (I/O), lpddr4_odt_120 (Input), lpddr4_odt_120_diff (Input), lpddr4_ocd_120p_120n (I/O), lpddr4_ocd_240p_240n (I/O), lpddr4_odt_240 (Input), lpddr4_ocd_40p_40n (I/O), lpddr4_odt_40 (Input), lpddr4_ocd_48p_48n (I/O), lpddr4_odt_48 (Input), lpddr4_ocd_60p_60n (I/O), lpddr4_odt_60 (Input), lpddr4_ocd_80p_80n (I/O), lpddr4_odt_80 (Input), lpddr4_odt_off (Input), lpddr4_ocd_120pd_60p_40n (I/O), lpddr4_ocd_120p_120n_diff (I/O), lpddr4_ocd_240p_240n_diff (I/O), lpddr4_odt_240_diff (Input), lpddr4_ocd_40p_40n_diff (I/O), lpddr4_odt_40_diff (Input), lpddr4_ocd_48p_48n_diff (I/O), lpddr4_odt_48_diff (Input), lpddr4_ocd_60p_60n_diff (I/O), lpddr4_odt_60_diff (Input), lpddr4_ocd_80p_80n_diff (I/O), lpddr4_ocd_120pd_60p_40n_diff (I/O), lpddr4_odt_80_diff (Input), lpddr4_odt_off_diff (Input), lpddr4_ocd_120pd_48p_40n (I/O), lpddr4_ocd_120pd_48p_40n_diff (I/O), emmc51_io_tx33ohm (I/O), emmc51_io_tx40ohm (I/O), emmc51_io_tx50ohm (I/O), emmc51_io_tx66ohm (I/O), emmc51_io_tx100ohm (I/O), emmc51_io_txod (I/O_open_drain), Cell18_0_0_H (I/O_open_drain), Cell18_0_1_H (I/O_open_drain), Cell18_0_2_H (I/O_open_drain), Cell18_0_3_H (I/O_open_drain)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
